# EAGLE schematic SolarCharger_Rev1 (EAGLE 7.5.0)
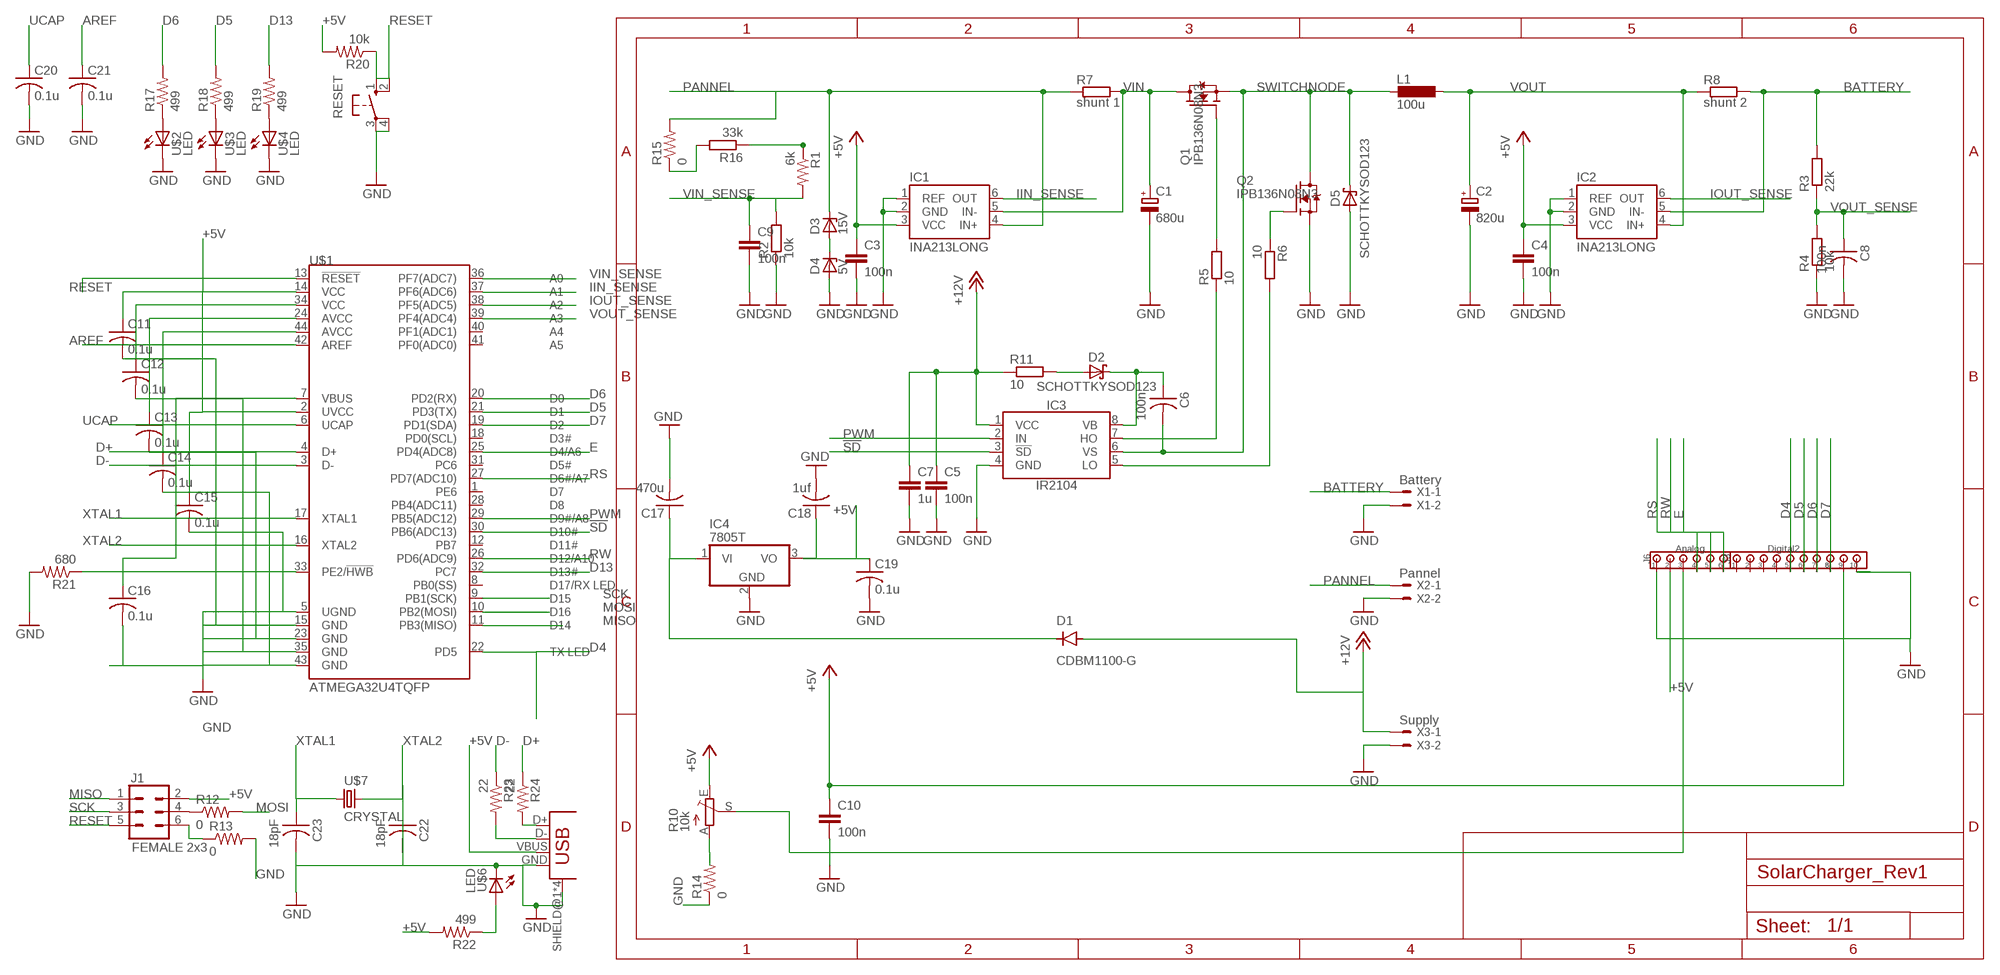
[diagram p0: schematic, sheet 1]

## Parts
C1  680u  C_POLARIZED10MM  [10MM]
C2  820u  C_POLARIZED10MM  [10MM]
C3  100n  CC0805  [C0805]
C4  100n  CC0805  [C0805]
C5  100n  CC0805  [C0805]
C6  100n  CAP-US1206FAB  [C1206FAB]
C7  1u  CC0805  [C0805]
C8  100n  CAP-US1206FAB  [C1206FAB]
C9  100n  CC0805  [C0805]
C10  100n  CC0805  [C0805]
C11  0.1u  C-USC1206  [C1206]
C12  0.1u  C-USC1206  [C1206]
C13  0.1u  C-USC1206  [C1206]
C14  0.1u  C-USC1206  [C1206]
C15  0.1u  C-USC1206  [C1206]
C16  0.1u  C-USC1206  [C1206]
C17  470u  C-USC1206  [C1206]
C18  1uf  C-USC1206  [C1206]
C19  0.1u  C-USC1206  [C1206]
C20  0.1u  C-USC1206  [C1206]
C21  0.1u  C-USC1206  [C1206]
C22  18pF  CAP-US1206FAB  [C1206FAB]
C23  18pF  CAP-US1206FAB  [C1206FAB]
D1  CDBM1100-G  [MINI-SMA]
D2  SCHOTTKYSOD123  [SOD123]
D3  15V  ZENER-DIODEZD-5  [ZDIO-5]
D4  5V  ZENER-DIODEZD-5  [ZDIO-5]
D5  SCHOTTKYSOD123  [SOD123]
IC1  INA213LONG  [SC70-6_LONG]
IC2  INA213LONG  [SC70-6_LONG]
IC3  IR2104  [SOIC8]
IC4  7805T  [TO220H]
J1  FEMALE 2x3  CONN_03X2FEMALE  [2X3]
J3  Digital2  100MIL_10X  [100MIL_10X_ROUND]
J6  Analog  100MIL_6X  [100MIL_6X_ROUND]
L1  100u  L-EU0207/12  [0207/12]
Q1  IPB136N08N3  N-PWR-MOSFETTO263-3  [TO263-3]
Q2  IPB136N08N3  IPB136N08N3_GTO263  [TO263-3@1]
R1  6k  RES-US1206FAB  [R1206FAB]
R2  10k  R-EU_M1206  [M1206]
R3  22k  R-EU_M1206  [M1206]
R4  10k  R-EU_M1206  [M1206]
R5  10  R-EU_M1206  [M1206]
R6  10  R-EU_M1206  [M1206]
R7  shunt 1  SMR  [SMR]
R8  shunt 2  SMR  [SMR]
R10  10k  TRIM_EU-B25X  [B25X]
R11  10  R-EU_M1206  [M1206]
R12  0  RES-US1206FAB  [R1206FAB]
R13  0  RES-US1206FAB  [R1206FAB]
R14  0  RES-US1206FAB  [R1206FAB]
R15  0  RES-US1206FAB  [R1206FAB]
R16  33k  R-EU_M1206  [M1206]
R17  499  RES-US1206  [R1206]
R18  499  RES-US1206  [R1206]
R19  499  RES-US1206  [R1206]
R20  10k  RES-US1206  [R1206]
R21  680  RES-US1206  [R1206]
R22  499  RES-US1206  [R1206]
R23  22  RES-US1206  [R1206]
R24  22  RES-US1206  [R1206]
RESET  10-XX  [B3F-10XX]
U$1  ATMEGA32U4TQFP  [SPARKFUN-DIGITALIC_TQFP44]
U$2  LED  [LED1206]
U$3  LED  [LED1206]
U$4  LED  [LED1206]
U$5  USB_MINIB  [USB_MINIB]
U$6  LED  [LED1206]
U$7  CRYSTAL  [2-SMD-5X3MM]
X1  Battery  22-23-2021200MIL  [200MIL_2X]
X2  Pannel  22-23-2021200MIL  [200MIL_2X]
X3  Supply  22-23-2021100MIL  [22-23-2021]

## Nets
!SD!: IC3.3(!SD!) U$1.30(PB6(ADC13))
+5V: C3.1 C4.1 C10.1 C11.1 C12.1 C13.1 C14.1 C15.1 C16.1 C18.1 C19.1 IC1.3(VCC) IC2.3(VCC) IC4.3(VO) J1.2 J6.2 R10.E R20.2 R22.2 U$1.2(UVCC) U$1.7(VBUS) U$1.14(VCC) U$1.24(AVCC) U$1.34(VCC) U$1.44(AVCC) U$5.VBUS
+12V: C5.1 C7.1 D1.ANODE IC3.1(VCC) R11.1 X3.1
AREF: C21.1 U$1.42(AREF)
BATTERY: IC2.5(IN-) R3.2 R8.1 X1.1
D4: J3.5 U$1.22(PD5)
D5: J3.6 R18.2 U$1.21(PD3(TX))
D6: J3.7 R17.2 U$1.20(PD2(RX))
D7: J3.8 U$1.19(PD1(SDA))
D13: R19.2 U$1.32(PC7)
D+: R24.1 U$1.4(D+)
D-: R23.1 U$1.3(D-)
E: J6.6 U$1.25(PD4(ADC8))
GND: C1.- C2.- C3.2 C4.2 C5.2 C7.2 C8.2 C9.2 C10.2 C11.2 C12.2 C13.2 C14.2 C15.2 C16.2 C17.2 C18.2 C19.2 C20.2 C21.2 C22.2 C23.2 D4.A D5.A IC1.1(REF) IC1.2(GND) IC2.1(REF) IC2.2(GND) IC3.4(GND) IC4.2(GND) J3.10 J6.1 Q2.3(S) R2.1 R4.1 R13.2 R14.1 R21.2 RESET.3(P) RESET.4(P1) U$1.5(UGND) U$1.15(GND) U$1.23(GND) U$1.35(GND) U$1.43(GND) U$2.2(C) U$3.2(C) U$4.2(C) U$5.GND U$5.SHIELD@1(SHIELD) U$5.SHIELD@2(SHIELD) U$5.SHIELD@3(SHIELD) U$5.SHIELD@4(SHIELD) U$6.2(C) X1.2 X2.2 X3.2
IIN_SENSE: IC1.6(OUT) U$1.37(PF6(ADC6))
IOUT_SENSE: IC2.6(OUT) U$1.38(PF5(ADC5))
MISO: J1.1 U$1.11(PB3(MISO))
MOSI: R12.2 U$1.10(PB2(MOSI))
N$1: J1.4 R12.1
N$2: J1.6 R13.1
N$3: R10.A R14.2
N$4: Q1.1(G) R5.2
N$5: R15.1 R16.2
N$7: Q2.1(G) R6.1
N$9: J3.9
N$10: J6.3 R10.S
N$11: D2.A R11.2
N$12: C6.1 D2.C IC3.8(VB)
N$14: IC3.7(HO) R5.1
N$15: IC3.5(LO) R6.2
N$17: R1.1 R16.1
N$19: D3.A D4.C
N$20: C17.1 D1.KATHODE IC4.1(VI)
N$21: R17.1 U$2.1(A)
N$22: R18.1 U$3.1(A)
N$23: R19.1 U$4.1(A)
N$24: R21.1 U$1.33(PE2/!HWB)
N$25: R24.2 U$5.D+
N$26: R22.1 U$6.1(A)
N$27: R23.2 U$5.D-
PANNEL: D3.C IC1.4(IN+) R7.2 R15.2 X2.1
PWM: IC3.2(IN) U$1.29(PB5(ADC12))
RESET: J1.5 R20.1 RESET.1(S) RESET.2(S1) U$1.13(!RESET)
RS: J6.4 U$1.27(PD7(ADC10))
RW: J6.5 U$1.26(PD6(ADC9))
SCK: J1.3 U$1.9(PB1(SCK))
SWITCHNODE: C6.2 D5.C IC3.6(VS) L1.2 Q1.3(S) Q2.TAB(D)
UCAP: C20.1 U$1.6(UCAP)
VIN: C1.+ IC1.5(IN-) Q1.TAB(D) R7.1
VIN_SENSE: C9.1 R1.2 R2.2 U$1.36(PF7(ADC7))
VOUT: C2.+ IC2.4(IN+) L1.1 R8.2
VOUT_SENSE: C8.1 R3.1 R4.2 U$1.39(PF4(ADC4))
XTAL1: C23.1 U$1.17(XTAL1) U$7.P$1
XTAL2: C22.1 U$1.16(XTAL2) U$7.P$2
Unconnected: J3.1 J3.2 J3.3 J3.4 U$1.1(PE6) U$1.8(PB0(SS)) U$1.12(PB7) U$1.18(PD0(SCL)) U$1.28(PB4(ADC11)) U$1.31(PC6) U$1.40(PF1(ADC1)) U$1.41(PF0(ADC0))

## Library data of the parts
C1 C2 = 00Capacitor:C_POLARIZED
C3-C5 C7 C9 C10 = 00Capacitor:C: Capacitor
C6 C8 C22 C23 = fab:CAP-US
C11-C21 = rcl:C-US: CAPACITOR, American symbol
D1 = fab:CDBM1100-G: Diode schottky 100V 1A mini-SMA as found in the fablab inventory
D2 D5 = 00Diode:SCHOTTKY
D3 D4 = diode:ZENER-DIODE: Z-Diode
IC1 IC2 = 00Sensor:INA21*: Current-Shunt Monitors Voltage Output, Low- or High-Side Measurement, Bidirectional, Zero-Drift Series; GAIN: 50
IC3 = 00Logic:IR2104: Half-Bridge Driver Up to +600V Gate drive supply 10-20V Deadtime 520ns
IC4 = linear:78*: Positive VOLTAGE REGULATOR Source: http://cache.national.com/ds/LM/LM78L05.pdf http://www.fairchildsemi.com/ds/LM/LM7805.pdf
J1 = SparkFun-Connectors:CONN_03X2: Multi connection point. Often used as Generic Header-pin footprint for 0.1 inch spaced/style header connections You can populate with any combo of single row headers, but if you'd like an exact match, check these: Header - 2x3 (Male, 0.1") (PRT-12807) Header - 2x3 (Female, 0.1") (PRT-13010) 2x3 Pin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; PROD_ID: CONN-11566
J3 = 00Connector:100MIL_10X: 100mil 10-pin connector
J6 = 00Connector:100MIL_6X: 100 mil 6-pin connector
L1 = rcl:L-EU: INDUCTOR, European symbol
Q1 = 00Mosfet:N-PWR-MOSFET
Q2 = 00Mosfet:IPB136N08N3_G
R1 R12-R15 R17-R24 = fab:RES-US: Resistor (US Symbol)
R2-R6 R11 R16 = rcl:R-EU_: RESISTOR, European symbol
R7 R8 = resistor-shunt:SMR: SMD SHUNT RESISTOR; OC_FARNELL: unknown; OC_NEWARK: unknown
R10 = pot:TRIM_EU-: POTENTIOMETER
RESET = switch-omron:10-XX: OMRON SWITCH; MPN: B3F-1000; OC_FARNELL: 176432; OC_NEWARK: 36M3542
U$1 = SparkFun-Retired:ATMEGA32U4: Atmel 44-pin 8-bit Microcontroller with 32KBytes of ISP Flash and USB Controller ----- Please use the QFN-44-NOPAD_1:1 package for the footprint of all boards using a 32U4. Route traces directly away from the pads as much as possible.; PROD_ID: IC-11161
U$2-U$4 U$6 = fab:LED: LED
U$5 = fab:USB_MINIB
U$7 = fab:CRYSTAL
X1 X2 = 00Connector:22-23-2021: .100" (2.54mm) Center Header - 2 Pin
X3 = 00Connector:22-23-2021: .100" (2.54mm) Center Header - 2 Pin; MF: MOLEX; MPN: 22-23-2021; OC_FARNELL: 1462926; OC_NEWARK: 25C3832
